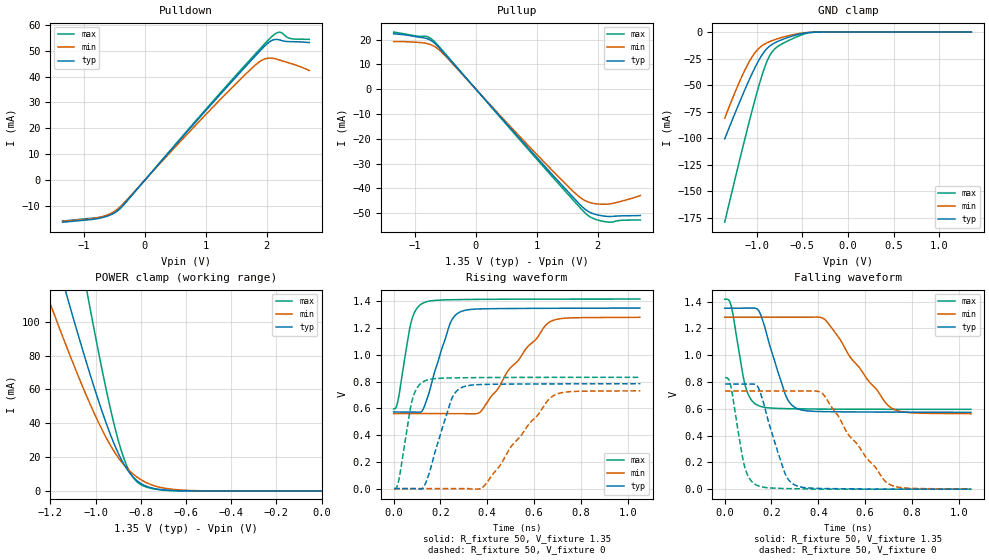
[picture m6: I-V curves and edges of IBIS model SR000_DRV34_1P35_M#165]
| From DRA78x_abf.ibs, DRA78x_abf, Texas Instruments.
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| Model based on original model for DDR_SEIOPB_V
|   Sub model SR000_DRV34_1P35
[model]   SR000_DRV34_1P35_M#165
|[Description]  [1.35V-I/O-X-X]
|   , ,
|[Input Load]
|[Output Drive]
|Voltage   1.35V
|Mode   I/O
Model_type   I/O
Polarity   Non-Inverting
Enable   Active-Low
Vinl =  0.585
Vinh =  0.765
Cref =  15.0000pF
Rref =  100.0000M
Vref =  0V
Vmeas =  0.675
C_comp   2p   2p   2p
[Model Spec]
Vinl   0.585   0.55125   0.61875
Vinh   0.765   0.73125   0.79875
[Receiver Thresholds]
Tslew_ac = 5n
Vth = 0.675
Vth_max = 0.709
Vth_min = 0.608
Vinh_ac = 0.175
Vinh_dc = 0.1
Vinl_ac = -0.175
Vinl_dc = -0.1
[Temperature Range]   25   125   -40
[Voltage Range]   1.35   1.2825   1.4175
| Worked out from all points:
|   slope of the pulldown table from 0 to 0.203 V, typ, clamps not added: 36.8 ohm
|   slope of the pullup table from 0 to 0.203 V, typ, clamps not added: 36 ohm
|   GND clamp passes 1 mA (typ) near -0.48 V on its own axis
|   POWER clamp passes 1 mA (typ) near -0.72 V on its own axis
|   rising waveform, R_fixture 50, V_fixture 1.35: 20-80 % time 79.9ps typ, 193ps min, 47.3ps max; typ from 0.573 V to 1.35 V
|   rising waveform, R_fixture 50, V_fixture 0: 20-80 % time 79.7ps typ, 187ps min, 47.6ps max; typ from 0 V to 0.784 V
|   falling waveform, R_fixture 50, V_fixture 1.35: 20-80 % time 80.9ps typ, 179ps min, 49.6ps max; typ from 1.35 V to 0.573 V
|   falling waveform, R_fixture 50, V_fixture 0: 20-80 % time 80.8ps typ, 183ps min, 48.8ps max; typ from 0.784 V to 0 V
[POWER_clamp]
-1.35V    224.4mA    165.8mA    358.5mA
-1.214V   157mA      115.5mA    250.8mA
-1.132V   117.8mA    86.59mA    187.7mA
-1.118V   111.4mA    81.92mA    177.3mA
-1.036V   74.26mA    55.16mA    116.8mA
-954.5mV  40.7mA     31.91mA    61.06mA
-900mV    22.42mA    19.79mA    30.14mA
-859.1mV  12.48mA    13.09mA    13.96mA
-804.5mV  4.85mA     7.084mA    4.132mA
-736.4mV  1.313mA    2.9mA      1.073mA
-627.3mV  101.6uA    577.3uA    45.9uA
0V        75.63nA    322.4nA    418.5nA
[Pulldown]
-1.35V    -16.25mA   -15.93mA   -15.81mA
-736.4mV  -14.67mA   -14.31mA   -14.33mA
-531.8mV  -13.09mA   -12.54mA   -12.91mA
-409.1mV  -10.94mA   -10.36mA   -11.07mA
1.145V    30.69mA    28.89mA    31.23mA
1.718V    45.54mA    42.37mA    46.27mA
1.923V    50.72mA    46.33mA    51.51mA
2.086V    53.98mA    47.12mA    55.52mA
2.209V    54.19mA    46.41mA    57.19mA
2.25V     53.89mA    46.1mA     56.9mA
2.373V    53.5mA     45.23mA    54.8mA
2.7V      53.13mA    42.33mA    54.36mA
[Pullup]
-1.35V    22.33mA    19.2mA     23.01mA
-981.8mV  21.15mA    18.91mA    21.43mA
-818.2mV  20.5mA     18.48mA    21.31mA
-736.4mV  19.62mA    17.88mA    20.36mA
-613.6mV  16.97mA    16.06mA    17.42mA
1.064V    -29.25mA   -27.93mA   -29.99mA
1.555V    -42.46mA   -40.17mA   -43.52mA
1.759V    -47.7mA    -44.45mA   -49.03mA
1.923V    -50.14mA   -45.98mA   -52.07mA
2.127V    -51.21mA   -46.35mA   -53.42mA
2.291V    -51.16mA   -45.77mA   -53.24mA
2.7V      -50.91mA   -42.85mA   -52.71mA
[GND_clamp]
-1.35V    -100.7mA   -81.27mA   -179.3mA
-1.241V   -77.31mA   -57.61mA   -140mA
-1.132V   -54.83mA   -36.31mA   -101.6mA
-1.05V    -39.08mA   -23.36mA   -74mA
-968.2mV  -25.28mA   -14.71mA   -48.34mA
-913.6mV  -18.13mA   -11.32mA   -33.52mA
-859.1mV  -13.28mA   -9.024mA   -22.35mA
-831.8mV  -11.61mA   -8.091mA   -18.64mA
-777.3mV  -9.078mA   -6.444mA   -14.07mA
-531.8mV  -1.871mA   -1.307mA   -3.441mA
-368.2mV  -88.76uA   -111.2uA   -158uA
1.35V     75.63nA    385.5nA    349.4nA
[Ramp]
dV/dt_f 0.46672581/80.98643p  0.43371359/0.1799224n  0.4936245/49.586613p
dV/dt_r 0.47316769/80.089995p  0.4421251/0.18889262n 0.50191117/47.824225p
R_load = 50
[Rising Waveform]
R_fixture = 50
V_fixture = 1.35
V_fixture_min = 1.2825
V_fixture_max = 1.4175
0s        573.3mV    561.4mV    596.6mV
19.73ps   572.6mV    561.3mV    668.6mV
76.21ps   572.5mV    561.3mV    1.255V
126.9ps   596.4mV    561.3mV    1.389V
238.7ps   1.223V     561.1mV    1.412V
283.1ps   1.321V     560.7mV    1.414V
372.3ps   1.344V     576.9mV    1.415V
492.7ps   1.347V     890.6mV    1.417V
670.8ps   1.349V     1.25V      1.417V
1.053ns   1.35V      1.282V     1.417V
[Rising Waveform]
R_fixture = 50
V_fixture = 0
V_fixture_min = 0
V_fixture_max = 0
1.843ps   0V         0V         0V
23.16ps   0V         0V         72.51mV
81.24ps   0V         0V         674.1mV
131ps     20.3mV     0V         803.7mV
244.7ps   657mV      0V         827.7mV
291.6ps   756.8mV    0V         829.1mV
385.3ps   779.2mV    17.14mV    830.5mV
504.8ps   781.7mV    320.7mV    831.4mV
684.2ps   783.2mV    696.2mV    831.9mV
1.054ns   784.4mV    732.7mV    832.1mV
[Falling Waveform]
R_fixture = 50
V_fixture = 1.35
V_fixture_min = 1.2825
V_fixture_max = 1.4175
0s        1.35V      1.282V     1.417V
28.93ps   1.35V      1.283V     1.359V
91.54ps   1.35V      1.283V     749.3mV
141.9ps   1.34V      1.283V     625.1mV
259.3ps   706.2mV    1.283V     600.8mV
306.2ps   604.1mV    1.282V     599.4mV
429.7ps   578.2mV    1.263V     597.3mV
538.7ps   576.2mV    979.5mV    596.5mV
715.5ps   574.6mV    602.3mV    595.9mV
1.053ns   573.3mV    561.4mV    595.7mV
[Falling Waveform]
R_fixture = 50
V_fixture = 0
V_fixture_min = 0
V_fixture_max = 0
1.843ps   784.4mV    732.7mV    832.1mV
26.83ps   784.6mV    732.8mV    764.8mV
86.79ps   784mV      732.8mV    158.2mV
138.6ps   771.5mV    732.8mV    28.43mV
255.6ps   126.8mV    732.8mV    4.702mV
301.4ps   29.67mV    732.5mV    3.16mV
419.4ps   4.884mV    710.8mV    0V
528.3ps   2.682mV    408mV      0V
702.9ps   0V         37.15mV    0V
1.054ns   0V         0V         0V
